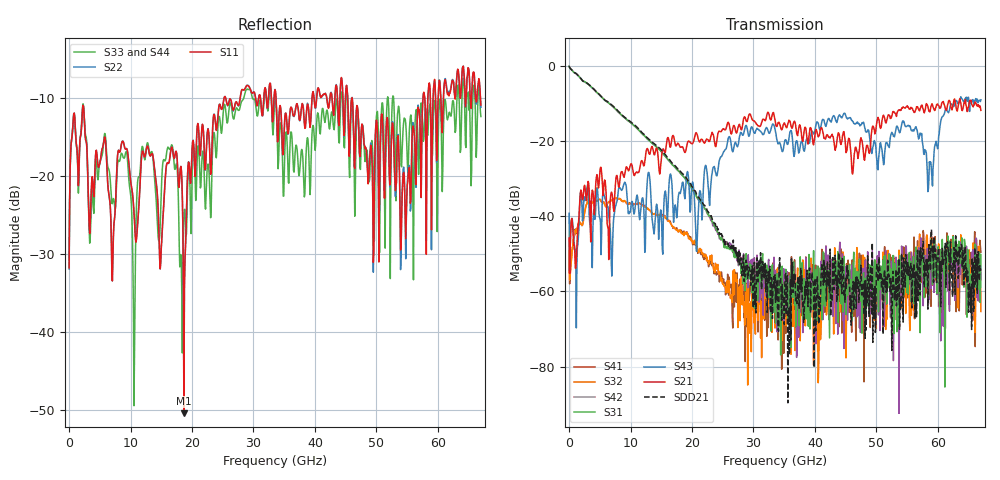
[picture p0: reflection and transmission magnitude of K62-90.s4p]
!Agilent Technologies,N5247A,US50470101,A.10.25.02
!Agilent N5247A: A.10.25.02
!Date: Tuesday, May 12, 2015 13:46:02
!Correction: Sdd11(Full 4 Port(1,2,3,4))
!Sdc11(Full 4 Port(1,2,3,4))
!Sdd12(Full 4 Port(1,2,3,4))
!Sdc12(Full 4 Port(1,2,3,4))
!Scd11(Full 4 Port(1,2,3,4))
!Scc11(Full 4 Port(1,2,3,4))
!Scd12(Full 4 Port(1,2,3,4))
!Scc12(Full 4 Port(1,2,3,4))
!Sdd21(Full 4 Port(1,2,3,4))
!Sdc21(Full 4 Port(1,2,3,4))
!Sdd22(Full 4 Port(1,2,3,4))
!Sdc22(Full 4 Port(1,2,3,4))
!Scd21(Full 4 Port(1,2,3,4))
!Scc21(Full 4 Port(1,2,3,4))
!Scd22(Full 4 Port(1,2,3,4))
!Scc22(Full 4 Port(1,2,3,4))
!Balanced Topology: BBAL
!S4P File: Measurements: <Sdd11,Sdc11,Sdd12,Sdc12>,
!<Scd11,Scc11,Scd12,Scc12>,
!<Sdd21,Sdc21,Sdd22,Sdc22>,
!<Scd21,Scc21,Scd22,Scc22>:
# Hz S  dB  R 50
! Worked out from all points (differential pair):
!   801 points, 10 MHz to 67 GHz, reference 50 ohm
!   strongest paths, dB at 10 MHz, 16.76 GHz, 33.51 GHz, 50.25 GHz, 67 GHz:
!     S21: -45.8, -19.1, -14.4, -13.7, -11.8
!     S43: -39.2, -31.9, -16.9, -27.7, -9.1
!     S31: -0.1, -26.2, -58.4, -53.5, -50.2
!     S42: -0.1, -26.2, -56.9, -61.1, -56.9
!     S32: -49.2, -42.7, -69.7, -59.6, -65.3
!     S41: -51.8, -42.7, -57.1, -56.8, -49.6
!   taken as a pair (ports 1,2 in; 3,4 out), SDD21 dB: -0.1, -25.8, -55.6, -57.4, -54.4
!   lowest |S11| = -50.4 dB at 18.68 GHz (marker M1), VSWR 1.01, Z = 50 - j0.302 ohm
!   |S11| at or under -10 dB: start of sweep to 25.25 GHz; 33.66 GHz to 39.54 GHz (5.879 GHz wide, 16.1 % of centre); 45.33 GHz to 57.6 GHz (12.28 GHz wide, 23.9 % of centre)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
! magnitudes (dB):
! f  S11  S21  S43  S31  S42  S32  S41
! 10 MHz  -31.8  -45.8  -39.2  -0.1  -0.1  -49.2  -51.8
! 4.364 GHz  -16.8  -31.0  -36.7  -6.9  -6.9  -35.8  -35.8
! 18.68 GHz  -50.4  -22.4  -33.1  -29.6  -29.5  -45.2  -44.0
! 28.98 GHz  -8.5  -14.8  -16.7  -52.6  -52.5  -59.4  -59.1
! 37.19 GHz  -11.1  -18.6  -20.9  -63.1  -58.4  -53.8  -65.9
! 58.71 GHz  -8.6  -12.3  -26.1  -52.0  -53.3  -50.6  -50.2
! 67 GHz  -11.0  -11.8  -9.1  -50.2  -56.9  -65.3  -49.6
